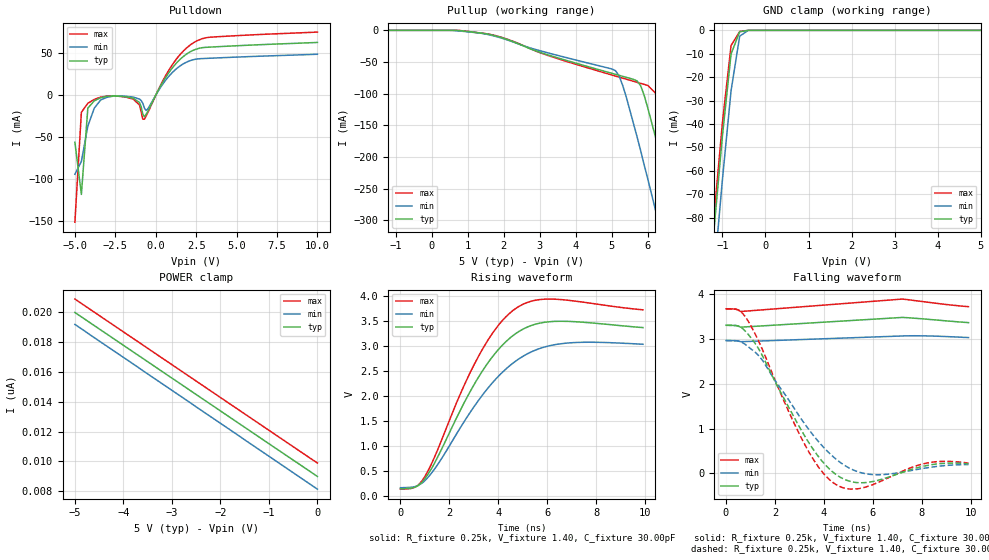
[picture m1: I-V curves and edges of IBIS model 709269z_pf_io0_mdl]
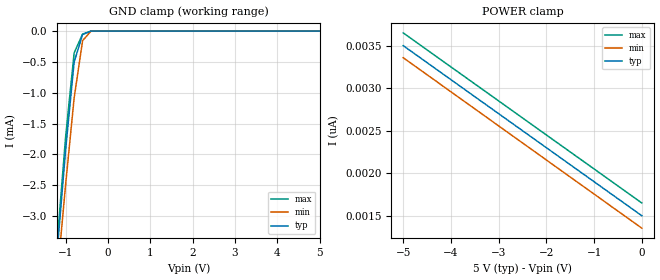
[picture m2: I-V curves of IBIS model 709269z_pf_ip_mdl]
| IBIS file 709269pf.ibs created by s2ibis2 version 1.0
| North Carolina State University Electronics Research Laboratory  1995
[IBIS ver]   2.1
[File name]   709269pf.ibs
[File Rev]   2.0
[Date]   06/15/97
[Source]   Integrated Device Technology, Inc.
[Notes]   1.Temperatures: typ=25C, min=100C, max=0C 2.Cemos8_5v process.
   3.RRmp rates based on 50 ohm load.
[Disclaimer]   This information is for modeling purpose only, and is not
   guaranteed.
[Copyright]   Copyright 1997, Integrated Device Technology, Inc. all rights
   reserved
|   Component 709269pf
[Component]   709269pf
[Manufacturer]   Integrated Device Technology
[Package]
| variable   typ   min   max
R_pkg   100.00m   90.00m   0.11
L_pkg   4.50nH   3.50nH   5.50nH
C_pkg   0.72pF   0.62pF   0.82pF
[Pin]  signal_name   model_name   R_pin   L_pin   C_pin
1   A9L   709269z_pf_ip_mdl
2   A10L   709269z_pf_ip_mdl
3   A11L   709269z_pf_ip_mdl
4   A12L   709269z_pf_ip_mdl
5   A13L   709269z_pf_ip_mdl
6   NC   NC
7   NC   NC
8   NC   NC
9   NC   NC
10   LBL   709269z_pf_ip_mdl
11   UBL   709269z_pf_ip_mdl
12   CE0BL   709269z_pf_ip_mdl
13   CE1L   709269z_pf_ip_mdl
14   CNTRSTBL   709269z_pf_ip_mdl
15   VCC   POWER
16   RWBL   709269z_pf_ip_mdl
17   OEBL   709269z_pf_ip_mdl
18   VCC   POWER
19   GND   GND
20   IO15L   709269z_pf_io0_mdl
21   IO14L   709269z_pf_io0_mdl
22   IO13L   709269z_pf_io0_mdl
23   IO12L   709269z_pf_io0_mdl
24   IO11L   709269z_pf_io0_mdl
25   IO10L   709269z_pf_io0_mdl
26   IO9L   709269z_pf_io0_mdl
27   IO8L   709269z_pf_io0_mdl
28   VCC   POWER
29   IO7L   709269z_pf_io0_mdl
30   IO6L   709269z_pf_io0_mdl
31   IO5L   709269z_pf_io0_mdl
32   IO4L   709269z_pf_io0_mdl
33   IO3L   709269z_pf_io0_mdl
34   IO2L   709269z_pf_io0_mdl
35   GND   GND
36   IO1L   709269z_pf_io0_mdl
37   IO0L   709269z_pf_io0_mdl
38   GND   GND
39   IO0R   709269z_pf_io0_mdl
40   IO1R   709269z_pf_io0_mdl
41   IO2R   709269z_pf_io0_mdl
42   IO3R   709269z_pf_io0_mdl
43   IO4R   709269z_pf_io0_mdl
44   IO5R   709269z_pf_io0_mdl
45   IO6R   709269z_pf_io0_mdl
46   VCC   POWER
47   IO7R   709269z_pf_io0_mdl
48   IO8R   709269z_pf_io0_mdl
49   IO9R   709269z_pf_io0_mdl
50   NC   NC
51   IO10R   709269z_pf_io0_mdl
52   IO11R   709269z_pf_io0_mdl
53   IO12R   709269z_pf_io0_mdl
54   IO13R   709269z_pf_io0_mdl
55   IO14R   709269z_pf_io0_mdl
56   IO15R   709269z_pf_io0_mdl
57   GND   GND
58   FT/PIPEBR   709269z_pf_ip_mdl
59   OEBR   709269z_pf_ip_mdl
60   RWBR   709269z_pf_ip_mdl
61   GND   GND
62   CNTRSTBR   709269z_pf_ip_mdl
63   CE1R   709269z_pf_ip_mdl
64   CEB0R   709269z_pf_ip_mdl
65   UBR   709269z_pf_ip_mdl
66   LBR   709269z_pf_ip_mdl
67   NC   NC
68   NC   NC
69   NC   NC
70   NC   NC
71   A13R   709269z_pf_ip_mdl
72   A12R   709269z_pf_ip_mdl
73   A11R   709269z_pf_ip_mdl
74   A10R   709269z_pf_ip_mdl
75   A9R   709269z_pf_ip_mdl
76   A8R   709269z_pf_ip_mdl
77   A7R   709269z_pf_ip_mdl
78   A6R   709269z_pf_ip_mdl
79   A5R   709269z_pf_ip_mdl
80   A4R   709269z_pf_ip_mdl
81   A3R   709269z_pf_ip_mdl
82   A2R   709269z_pf_ip_mdl
83   A1R   709269z_pf_ip_mdl
84   A0R   709269z_pf_ip_mdl
85   CNTENBR   709269z_pf_ip_mdl
86   CLKR   709269z_pf_ip_mdl
87   ADSBR   709269z_pf_ip_mdl
88   GND   GND
89   ADSBL   709269z_pf_ip_mdl
90   CLKL   709269z_pf_ip_mdl
91   CNTENBL   709269z_pf_ip_mdl
92   A0L   709269z_pf_ip_mdl
93   A1L   709269z_pf_ip_mdl
94   A2L   709269z_pf_ip_mdl
95   A3L   709269z_pf_ip_mdl
96   A4L   709269z_pf_ip_mdl
97   A5L   709269z_pf_ip_mdl
98   A6L   709269z_pf_ip_mdl
99   A7L   709269z_pf_ip_mdl
100   A8L   709269z_pf_ip_mdl
| Models and submodels in the file (2): 709269z_pf_io0_mdl (I/O), 709269z_pf_ip_mdl (Input)
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| in0  in0   dummy_model
| oel0 oel0   dummy_model
| in1  in1   dummy_model
| oel1 oel1   dummy_model
| in2  in2   dummy_model
| oel2 oel2   dummy_model
|   Model 709269z_pf_io0_mdl
[Model]   709269z_pf_io0_mdl
Model_type   I/O
Polarity   Non-Inverting
Enable   Active-High
Vinl =  0.800V
Vinh =  2.000V
Vmeas =  1.500V
C_comp   3.00pF   NA   NA
[Temperature Range]   25.00   100.00   0.000
[Voltage Range]   5.00V   4.50V   5.50V
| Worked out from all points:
|   slope of the pulldown table from 0 to 0.75 V, typ, clamps not added: 29.8 ohm
|   slope of the pullup table from 0 to 0.75 V, typ, clamps not added: 1.9 kohm
|   GND clamp passes 1 mA (typ) near -0.61 V on its own axis
|   rising waveform, R_fixture 0.25k, V_fixture 1.40, C_fixture 30.00pF: 20-80 % time 2.13ns typ, 2.47ns min, 1.98ns max; typ from 0.136 V to 3.37 V
|   falling waveform, R_fixture 0.25k, V_fixture 1.40, C_fixture 30.00pF: 20-80 % time 1.07ns typ, 2.04ns min, NA max; typ from 3.31 V to 3.37 V
|   falling waveform, R_fixture 0.25k, V_fixture 1.40, C_fixture 30.00pF: 20-80 % time 1.79ns typ, 2.09ns min, 1.65ns max; typ from 3.31 V to 0.217 V
[Pulldown]
| voltage   I(typ)   I(min)   I(max)
-5V       -56mA      -94mA      -151mA
-4.6V     -118mA     -78.9mA    -20.4mA
-4.2V     -15.4mA    -36.8mA    -9.6mA
-3.8V     -6.7mA     -15.4mA    -5mA
-3V       -1.3mA     -2.5mA     -1mA
-1.4V     -3.6mA     -2.2mA     -4.6mA
-1V       -8.71mA    -4.73mA    -11.79mA
-700mV    -25.54mA   -15.32mA   -28.54mA
-500mV    -19.47mA   -16.55mA   -21.27mA
1V        31.71mA    26.39mA    35.42mA
2.5V      54.67mA    42.84mA    64.08mA
10V       62.67mA    48.64mA    74.98mA
[Pullup]
| voltage   I(typ)   I(min)   I(max)
-5V       -3.99nA    -3.59nA    -4.39nA
1.1V      -2.523mA   -2.891mA   -2.378mA
5V        -67.81mA   -60.96mA   -70.47mA
5.2V      -70.97mA   -71.52mA   -73.79mA
5.3V      -72.55mA   -86.72mA   -75.45mA
5.8V      -87.42mA   -190mA     -83.7mA
6V        -123mA     -235mA     -86.99mA
6.4V      -209mA     -327mA     -110mA
6.8V      -301mA     -421mA     -192mA
7.2V      -395mA     -519mA     -284mA
7.6V      -491mA     -617mA     -378mA
10V       -1.098A    -1.191A    -1A
[GND_clamp]
| voltage   I(typ)   I(min)   I(max)
-5V       -1.041A    -993mA     -1.025A
-1.4V     -128mA     -147mA     -123mA
-1.2V     -85.73mA   -105mA     -80.04mA
-1V       -44.9mA    -63.57mA   -39.23mA
-800mV    -10.12mA   -25.76mA   -6.522mA
-600mV    -613uA     -2.497mA   -513uA
-400mV    -12.16nA   -4.645uA   -3.686nA
5V        8.994nA    9.245nA    8.794nA
[POWER_clamp]
| voltage   I(typ)   I(min)   I(max)
-5V       19.99nA    19.19nA    20.89nA
-4.7V     19.33nA    18.52nA    20.23nA
-3.7V     17.13nA    16.32nA    18.03nA
0V        8.994nA    8.141nA    9.894nA
[Ramp]
| variable   typ   min   max
dV/dt_r   1.11/1.58n   0.93/1.73n   1.27/1.46n
dV/dt_f   1.60/1.95n   1.27/2.15n   1.88/1.85n
R_load = 50.00
[Rising Waveform]
R_fixture = 0.25k
V_fixture = 1.40
C_fixture = 30.00pF
R_dut = 100.00m
L_dut = 4.50nH
C_dut = 0.72pF
| time   V(typ)   V(min)   V(max)
0s        136mV      156mV      127mV
600ps     169mV      179mV      167mV
1ns       337mV      298mV      383mV
2.5ns     1.762V     1.402V     2.097V
3.2ns     2.382V     1.915V     2.802V
4ns       2.926V     2.39V      3.413V
4.6ns     3.207V     2.655V     3.711V
5.4ns     3.417V     2.891V     3.902V
6.4ns     3.491V     3.031V     3.932V
9.9ns     3.365V     3.031V     3.721V
[Falling Waveform]
R_fixture = 0.25k
V_fixture = 1.40
C_fixture = 30.00pF
R_dut = 100.00m
L_dut = 4.50nH
C_dut = 0.72pF
| time   V(typ)   V(min)   V(max)
0s        3.306V     2.965V     3.674V
300ps     3.303V     2.963V     3.67V
400ps     3.3V       2.961V     3.664V
500ps     3.288V     2.955V     3.648V
600ps     3.263V     2.939V     3.613V
7.2ns     3.481V     3.067V     3.891V
7.7ns     3.463V     3.072V     3.858V
8.1ns     3.446V     3.07V      3.83V
9ns       3.404V     3.054V     3.769V
9.9ns     3.365V     3.031V     3.721V
[Falling Waveform]
R_fixture = 0.25k
V_fixture = 1.40
C_fixture = 30.00pF
R_dut = 100.00m
L_dut = 4.50nH
C_dut = 0.72pF
| time   V(typ)   V(min)   V(max)
0s        3.306V     2.965V     3.674V
500ps     3.288V     2.955V     3.648V
900ps     3.107V     2.831V     3.404V
1.5ns     2.613V     2.516V     2.75V
3.2ns     848mV      1.114V     661mV
4.4ns     13.61mV    360mV      -218mV
5.1ns     -184mV     99.03mV    -351mV
6ns       -181mV     -27.7mV    -250mV
8.1ns     164mV      115mV      218mV
9.9ns     217mV      196mV      229mV
|   Model 709269z_pf_ip_mdl
[Model]   709269z_pf_ip_mdl
Model_type   Input
Vinl =  0.800V
Vinh =  2.000V
Vmeas =  1.500V
C_comp   3.00pF   NA   NA
[Temperature Range]   25.00   100.00   0.000
[Voltage Range]   5.00V   4.50V   5.50V
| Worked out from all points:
|   GND clamp passes 1 mA (typ) near -0.87 V on its own axis
[GND_clamp]
| voltage   I(typ)   I(min)   I(max)
-5V       -37.62mA   -34.5mA    -38.75mA
-1.2V     -3.576mA   -3.985mA   -3.42mA
-1V       -1.917mA   -2.481mA   -1.707mA
-800mV    -503uA     -1.086mA   -355uA
-600mV    -54.94uA   -155uA     -48.04uA
-400mV    -1.068nA   -216nA     -734pA
5V        1.5nA      1.554nA    1.45nA
[POWER_clamp]
| voltage   I(typ)   I(min)   I(max)
-5V       3.5nA      3.358nA    3.65nA
-800mV    1.82nA     1.675nA    1.97nA
-700mV    1.78nA     1.634nA    1.93nA
0V        1.5nA      1.354nA    1.65nA
